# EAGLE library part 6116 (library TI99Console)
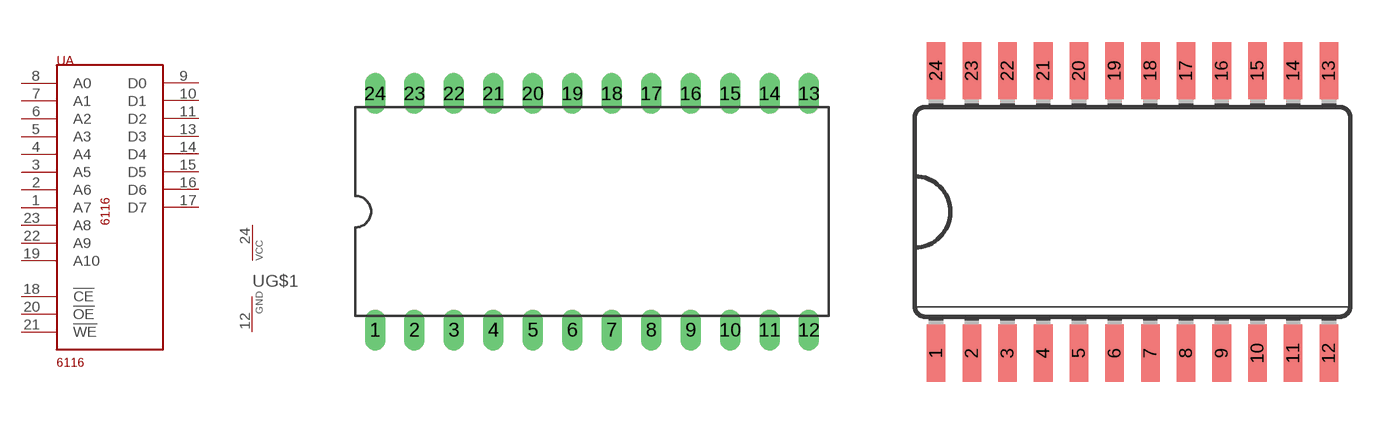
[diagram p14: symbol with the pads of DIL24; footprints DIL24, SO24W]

Designator prefix -; gates G$1=VCC-GND A=6116

## 6116DIL24  [DIL24]
1  A:A7  in
2  A:A6  in
3  A:A5  in
4  A:A4  in
5  A:A3  in
6  A:A2  in
7  A:A1  in
8  A:A0  in
9  A:D0
10  A:D1
11  A:D2
12  G$1:GND  pwr
13  A:D3
14  A:D4
15  A:D5
16  A:D6
17  A:D7
18  A:!CE  in
19  A:A10  in
20  A:!OE  in
21  A:!WE  in
22  A:A9  in
23  A:A8  in
24  G$1:VCC  pwr

## 6116SO24W  [SO24W]
Pads as for DIL24

## Footprint DIL24 (pad centres in mm)
Dual In Line Package
drill 0.813 long: 1 -13.97,-7.62; 2 -11.43,-7.62; 3 -8.89,-7.62; 4 -6.35,-7.62; 5 -3.81,-7.62; 6 -1.27,-7.62; 7 1.27,-7.62; 8 3.81,-7.62; 9 6.35,-7.62; 10 8.89,-7.62; 11 11.43,-7.62; 12 13.97,-7.62; 13 13.97,7.62; 14 11.43,7.62; 15 8.89,7.62; 16 6.35,7.62; 17 3.81,7.62; 18 1.27,7.62; 19 -1.27,7.62; 20 -3.81,7.62; 21 -6.35,7.62; 22 -8.89,7.62; 23 -11.43,7.62; 24 -13.97,7.62

## Footprint SO24W (pad centres in mm)
Wide Small Outline package 300 mil
smd 0.66 x 2.032: 1 -6.985,-5.029; 2 -5.715,-5.029; 3 -4.445,-5.029; 4 -3.175,-5.029; 5 -1.905,-5.029; 6 -0.635,-5.029; 7 0.635,-5.029; 8 1.905,-5.029; 9 3.175,-5.029; 10 4.445,-5.029; 11 5.715,-5.029; 12 6.985,-5.029; 13 6.985,5.029; 14 5.715,5.029; 15 4.445,5.029; 16 3.175,5.029; 17 1.905,5.029; 18 0.635,5.029; 19 -0.635,5.029; 20 -1.905,5.029; 21 -3.175,5.029; 22 -4.445,5.029; 23 -5.715,5.029; 24 -6.985,5.029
